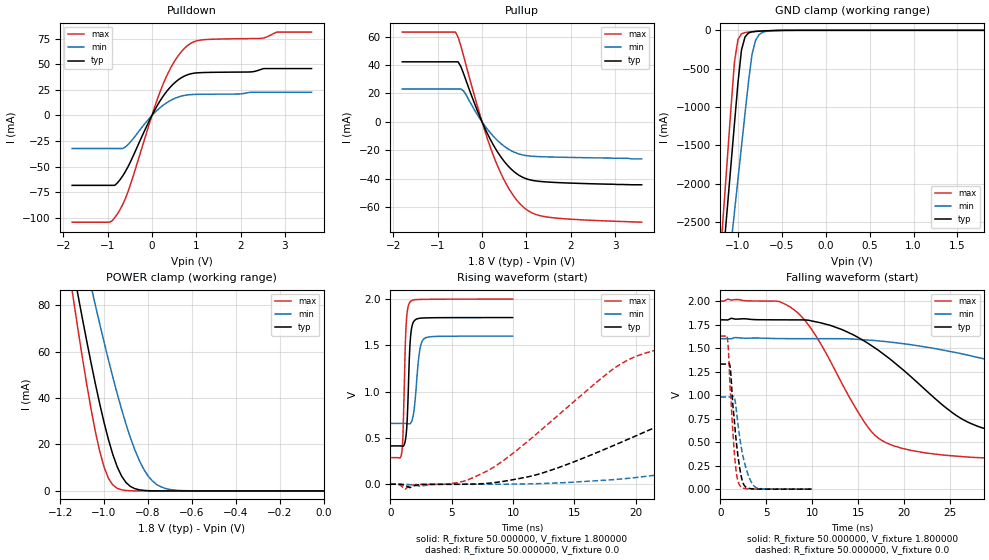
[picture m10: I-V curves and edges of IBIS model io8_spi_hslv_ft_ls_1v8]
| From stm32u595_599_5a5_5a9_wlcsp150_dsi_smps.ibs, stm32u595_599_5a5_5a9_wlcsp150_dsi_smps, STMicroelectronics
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|   Model io8_spi_hslv_ft_ls_1v8
[Model]  io8_spi_hslv_ft_ls_1v8
Model_type I/O
Polarity   Non-Inverting
Enable   Active-Low
Vinl =   0.540000V
Vinh =   1.260000V
Vmeas =  0.900000V
Cref =   50.000000pF
Rref =   100.000000M
Vref =   0.0V
C_comp   3.338700pF   3.332500pF   3.379000pF
[Temperature Range]   25.000000   0.140000k   -40.000000
[Pullup Reference]   1.800000V   1.600000V   2.000000V
[Pulldown Reference]   0.0V   0.0V   0.0V
[POWER Clamp Reference]   1.800000V   1.600000V   2.000000V
[GND Clamp Reference]   0.0V   0.0V   0.0V
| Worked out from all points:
|   slope of the pulldown table from 0 to 0.27 V, typ, clamps not added: 13.6 ohm
|   slope of the pullup table from 0 to 0.27 V, typ, clamps not added: 15.9 ohm
|   GND clamp passes 1 mA (typ) near -0.51 V on its own axis
|   POWER clamp passes 1 mA (typ) near -0.86 V on its own axis
|   rising waveform, R_fixture 50.000000, V_fixture 1.800000: 20-80 % time 238ps typ, 382ps min, 212ps max; typ from 0.414 V to 1.8 V
|   rising waveform, R_fixture 50.000000, V_fixture 0.0: 20-80 % time 15.2ns typ, 31.7ns min, 8.92ns max; typ from 0 V to 1.33 V
|   falling waveform, R_fixture 50.000000, V_fixture 1.800000: 20-80 % time 10.9ns typ, 26.4ns min, 6.09ns max; typ from 1.8 V to 0.414 V
|   falling waveform, R_fixture 50.000000, V_fixture 0.0: 20-80 % time 793ps typ, 1.07ns min, 618ps max; typ from 1.33 V to 0 V
[Pulldown]
|Voltage   I(typ)   I(min)   I(max)
-1.8V     -68.38mA   -32.32mA   -104.4mA
-960mV    -68.38mA   -32.32mA   -104.4mA
-780mV    -66.07mA   -32.32mA   -96.42mA
-540mV    -50.22mA   -28.51mA   -74.66mA
0V        0A         -700fA     0A
240mV     18.04mA    9.598mA    29.42mA
480mV     30.68mA    16.02mA    50.95mA
780mV     39.47mA    19.98mA    67.56mA
1.14V     41.99mA    20.77mA    74.01mA
2.46V     45.09mA    22.69mA    75.44mA
2.82V     45.91mA    22.69mA    81.6mA
3.6V      45.91mA    22.69mA    81.6mA
[Pullup]
|Voltage   I(typ)   I(min)   I(max)
-1.8V     42.21mA    23.08mA    63.11mA
-600mV    42.21mA    23.08mA    63.11mA
-540mV    42.21mA    23.08mA    59.57mA
-420mV    34.21mA    21.83mA    46.75mA
0V        630fA      250pA      10fA
300mV     -18.63mA   -11.6mA    -27.18mA
600mV     -31.41mA   -19.24mA   -46.67mA
780mV     -36.41mA   -22mA      -54.88mA
960mV     -39.54mA   -23.51mA   -60.64mA
1.2V      -41.44mA   -24.28mA   -64.94mA
1.56V     -42.42mA   -24.69mA   -67.24mA
3.6V      -44.2mA    -26mA      -70.5mA
[GND_clamp]
|Voltage   I(typ)   I(min)   I(max)
-1.8V     -9.908A    -9.683A    -9.994A
-1.2V     -3.383A    -4.084A    -2.934A
-1.16V    -2.841A    -3.655A    -2.294A
-1.12V    -2.299A    -3.226A    -1.656A
-1.04V    -1.218A    -2.369A    -414.2mA
-1V       -684.7mA   -1.941A    -119.2mA
-960mV    -257.2mA   -1.514A    -45.66mA
-920mV    -87.03mA   -1.089A    -28.93mA
-840mV    -19.35mA   -312.8mA   -18.96mA
-800mV    -13.55mA   -132.4mA   -15.49mA
-720mV    -8.042mA   -25.66mA   -9.49mA
1.8V      0A         13.64nA    0A
[POWER_clamp]
|Voltage   I(typ)   I(min)   I(max)
-1.8V     470.8mA    433.7mA    554.6mA
-1.14V    95.25mA    122.7mA    82.82mA
-1.12V    84.97mA    114mA      70.27mA
-1.06V    55.51mA    88.42mA    35.67mA
-1.04V    46.34mA    80.15mA    25.76mA
-1V       29.51mA    64.13mA    10.3mA
-940mV    10.39mA    41.86mA    1.109mA
-900mV    3.624mA    28.77mA    182.8uA
-840mV    490.7uA    13.24mA    11.35uA
-800mV    116.8uA    6.532mA    1.77uA
-740mV    13.2uA     1.724mA    109.3nA
0V        0A         18.75nA    0A
[Ramp]
| variable   typ   min   max
dV/dt_r  0.79770/15.20614n   0.58805/31.67983n   0.97668/8.90636n
dV/dt_f  0.83162/10.91511n   0.56540/26.37622n   1.02769/6.07445n
R_load = 50.000000
[Rising Waveform]
R_fixture= 50.000000
V_fixture= 1.800000
V_fixture_min= 1.600000
V_fixture_max= 2.000000
|time   V(typ)   V(min)   V(max)
0s        414mV      657mV      287.2mV
940.9ps   411.5mV    657mV      348mV
1.041ns   410.8mV    657.1mV    560.4mV
1.281ns   522.5mV    656.6mV    1.693V
1.401ns   766mV      654.6mV    1.882V
1.622ns   1.54V      655.4mV    1.97V
1.962ns   1.766V     826.5mV    1.992V
2.402ns   1.792V     1.448V     1.996V
2.763ns   1.796V     1.573V     1.997V
9.97ns    1.8V       1.6V       2V
[Rising Waveform]
R_fixture= 50.000000
V_fixture= 0.0
V_fixture_min= 0.0
V_fixture_max= 0.0
|time   V(typ)   V(min)   V(max)
0s        1.85nV     146.7nV    1.205nV
4.805ns   -866.2uV   -512.5uV   4.158mV
8.008ns   10.76mV    -25.73uV   151.4mV
12.41ns   121.8mV    7.751mV    599.8mV
20.02ns   523mV      72.87mV    1.381V
30.03ns   1.041V     265.6mV    1.579V
42.84ns   1.259V     535.3mV    1.619V
57.66ns   1.31V      775.4mV    1.627V
75.28ns   1.326V     905mV      1.628V
199.4ns   1.33V      980.3mV    1.628V
[Falling Waveform]
R_fixture= 50.000000
V_fixture= 1.800000
V_fixture_min= 1.600000
V_fixture_max= 2.000000
|time   V(typ)   V(min)   V(max)
0s        1.8V       1.6V       2V
7.608ns   1.8V       1.6V       1.936V
10.01ns   1.787V     1.6V       1.687V
16.82ns   1.502V     1.58V      573.2mV
24.42ns   875.1mV    1.475V     361.1mV
28.43ns   654.4mV    1.391V     333.9mV
34.83ns   536.4mV    1.225V     310.8mV
47.25ns   462.4mV    929.5mV    294.5mV
63.66ns   431mV      774.6mV    288.8mV
199.4ns   414mV      657mV      287.2mV
[Falling Waveform]
R_fixture= 50.000000
V_fixture= 0.0
V_fixture_min= 0.0
V_fixture_max= 0.0
|time   V(typ)   V(min)   V(max)
0s        1.33V      980.3mV    1.628V
760.8ps   1.329V     980.4mV    1.607V
880.9ps   1.335V     980.4mV    1.466V
1.081ns   1.28V      980.2mV    1.041V
1.542ns   702.2mV    969.9mV    363.3mV
1.782ns   458.3mV    799.8mV    145.1mV
2.082ns   237.3mV    564.9mV    44.14mV
2.623ns   37.04mV    280.7mV    7.416mV
3.844ns   1.771mV    19.03mV    1.16mV
9.97ns    1.85nV     146.7nV    1.205nV
